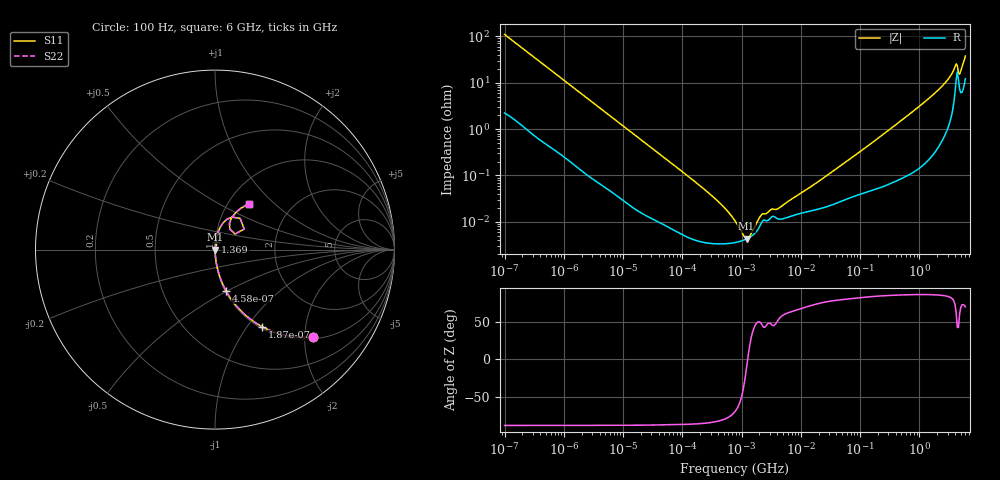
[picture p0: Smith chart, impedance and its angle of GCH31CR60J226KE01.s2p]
!Murata Part Number: GCH31CR60J226KE01
!These Parameters are Measured in Series Mode Connection
!Data Generated on Jun 19, 2026
!  o--ll--o
!Port1  Port2
!  o------o
!Operation Temp=25[degC], DC Bias Voltage=0[V]
!Freq. Start=100[Hz] Stop=6[GHz] 401[Steps]
# Hz S RI R 50
!Freq.(Hz) S11(Real) S11(Imag) S21(Real) S21(Imag) S12(Real) S12(Imag) S22(Real) S22(Imag)
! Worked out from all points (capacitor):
!   401 points, 100 Hz to 6 GHz, reference 50 ohm
!   read as one part in series: C = 14.4 uF near 109 Hz
!   lowest |Z| = 4.36 mohm at 1.212 MHz (marker M1)
!   series resonance near 1.266 MHz, so ESL is about 1.1 nH
!   S11 on the Smith chart (normalised r, x): 100 Hz: 1.04, -2.19; 187 Hz: 1.02, -1.18; 458 Hz: 1.01, -0.49; 1.369 GHz: 1.00, +0.09; 6 GHz: 1.24, +0.71
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100  0.5445 -0.488  0.4555 0.488  0.4555 0.488  0.5445 -0.488
187  0.2636 -0.4301  0.7364 0.4301  0.7364 0.4301  0.2636 -0.4301
280  0.1415 -0.3384  0.8585 0.3384  0.8585 0.3384  0.1415 -0.3384
458  0.0605 -0.2283  0.9395 0.2283  0.9395 0.2283  0.0605 -0.2283
897  0.0183 -0.1233  0.9817 0.1233  0.9817 0.1233  0.0183 -0.1233
2008  0.00446 -0.0566  0.9955 0.0566  0.9955 0.0566  0.00446 -0.0566
40335  0.000107 -0.00295  0.9999 0.00295  0.9999 0.00295  0.000107 -0.00295
316350  3.41e-05 -0.000362  1 0.000362  1 0.000362  3.41e-05 -0.000362
517687  3.37e-05 -0.000197  1 0.000197  1 0.000197  3.37e-05 -0.000197
774597  3.57e-05 -9.91e-05  1 9.91e-05  1 9.91e-05  3.57e-05 -9.91e-05
1212075  4.27e-05 -8.6e-06  1 8.6e-06  1 8.6e-06  4.27e-05 -8.6e-06
1734173  5.92e-05 6.4e-05  0.9999 -6.4e-05  0.9999 -6.4e-05  5.92e-05 6.4e-05
2268635  0.000105 0.000105  0.9999 -0.000105  0.9999 -0.000105  0.000105 0.000105
4246196  0.000115 0.00016  0.9999 -0.00016  0.9999 -0.00016  0.000115 0.00016
1.555665e7  0.000175 0.000573  0.9998 -0.000573  0.9998 -0.000573  0.000175 0.000573
3.124326e8  0.000746 0.00969  0.9993 -0.00969  0.9993 -0.00969  0.000746 0.00969
1.369159e9  0.00387 0.0428  0.9961 -0.0428  0.9961 -0.0428  0.00387 0.0428
2.679998e9  0.0161 0.0941  0.9839 -0.0941  0.9839 -0.0941  0.0161 0.0941
3.505958e9  0.0404 0.1425  0.9596 -0.1425  0.9596 -0.1425  0.0404 0.1425
4.009986e9  0.0942 0.181  0.9058 -0.181  0.9058 -0.181  0.0942 0.181
5.016141e9  0.0807 0.147  0.9193 -0.147  0.9193 -0.147  0.0807 0.147
6e9  0.1896 0.2554  0.8104 -0.2554  0.8104 -0.2554  0.1896 0.2554
